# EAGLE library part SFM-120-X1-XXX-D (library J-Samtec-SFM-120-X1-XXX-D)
0.05"X0.05" SOCKET STRIP DOUBLE ROW ASSEMBLY. MANUFACTURER: SAMTEC.
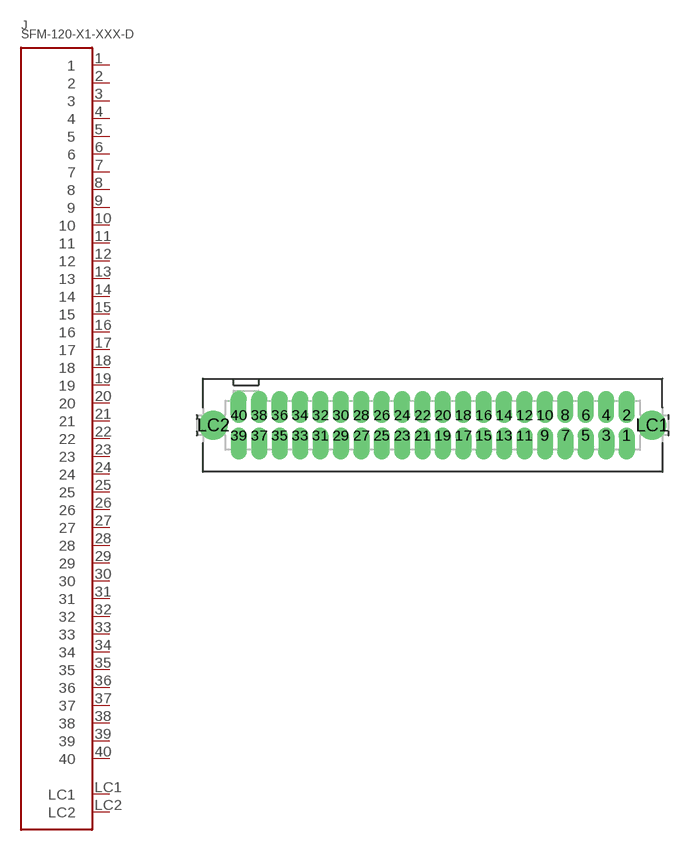
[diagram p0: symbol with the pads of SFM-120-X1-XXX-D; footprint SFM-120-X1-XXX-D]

Designator prefix J

## SFM-120-X1-XXX-D  [SFM-120-X1-XXX-D]
1  1  pas
2  2  pas
3  3  pas
4  4  pas
5  5  pas
6  6  pas
7  7  pas
8  8  pas
9  9  pas
10  10  pas
11  11  pas
12  12  pas
13  13  pas
14  14  pas
15  15  pas
16  16  pas
17  17  pas
18  18  pas
19  19  pas
20  20  pas
21  21  pas
22  22  pas
23  23  pas
24  24  pas
25  25  pas
26  26  pas
27  27  pas
28  28  pas
29  29  pas
30  30  pas
31  31  pas
32  32  pas
33  33  pas
34  34  pas
35  35  pas
36  36  pas
37  37  pas
38  38  pas
39  39  pas
40  40  pas
LC1  LC1  pas
LC2  LC2  pas

## Footprint SFM-120-X1-XXX-D (pad centres in mm)
0.05"X0.05" SOCKET STRIP DOUBLE ROW ASSEMBLY. MANUFACTURER: SAMTEC.
drill 0.5 offset: 1 12.065,-0.635; 2 12.065,0.635; 3 10.795,-0.635; 4 10.795,0.635; 5 9.525,-0.635; 6 9.525,0.635; 7 8.255,-0.635; 8 8.255,0.635; 9 6.985,-0.635; 10 6.985,0.635; 11 5.715,-0.635; 12 5.715,0.635; 13 4.445,-0.635; 14 4.445,0.635; 15 3.175,-0.635; 16 3.175,0.635; 17 1.905,-0.635; 18 1.905,0.635; 19 0.635,-0.635; 20 0.635,0.635; 21 -0.635,-0.635; 22 -0.635,0.635; 23 -1.905,-0.635; 24 -1.905,0.635; 25 -3.175,-0.635; 26 -3.175,0.635; 27 -4.445,-0.635; 28 -4.445,0.635; 29 -5.715,-0.635; 30 -5.715,0.635; 31 -6.985,-0.635; 32 -6.985,0.635; 33 -8.255,-0.635; 34 -8.255,0.635; 35 -9.525,-0.635; 36 -9.525,0.635; 37 -10.795,-0.635; 38 -10.795,0.635; 39 -12.065,-0.635; 40 -12.065,0.635
drill 1.194: LC1 13.652,0; LC2 -13.652,0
